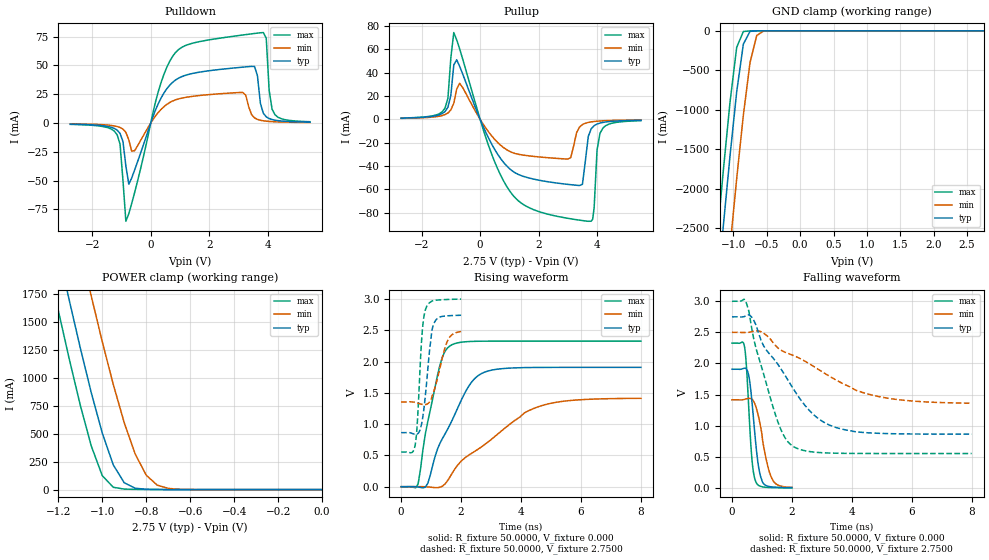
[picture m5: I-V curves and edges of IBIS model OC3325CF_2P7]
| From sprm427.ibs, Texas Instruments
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|   Model OC3325CF_2P7
[Model]   OC3325CF_2P7
Model_type   3-state
Polarity   Non-Inverting
Enable   Active-Low
Vmeas =   1.2500V
Cref =  15.0000pF
Rref = 100.0000M
Vref =  0.000V
C_comp   3.2189pF   3.2468pF   3.2081pF
[Temperature Range]   25.0000   0.1250k   -40.0000
[Pullup Reference]   2.7500V   2.5000V   3.0000V
[Pulldown Reference]   0.000V   0.000V   0.000V
[POWER Clamp Reference]   2.7500V   2.5000V   3.0000V
[GND Clamp Reference]   0.000V   0.000V   0.000V
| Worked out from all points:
|   slope of the pulldown table from 0 to 0.412 V, typ, clamps not added: 16.9 ohm
|   slope of the pullup table from 0 to 0.412 V, typ, clamps not added: 18.8 ohm
|   GND clamp passes 1 mA (typ) near -0.66 V on its own axis
|   POWER clamp passes 1 mA (typ) near -0.74 V on its own axis
|   rising waveform, R_fixture 50.0000, V_fixture 0.000: 20-80 % time 1.08ns typ, 2.21ns min, 559ps max; typ from 0 V to 1.91 V
|   rising waveform, R_fixture 50.0000, V_fixture 2.7500: 20-80 % time 237ps typ, 359ps min, 167ps max; typ from 0.864 V to 2.74 V
|   falling waveform, R_fixture 50.0000, V_fixture 0.000: 20-80 % time 236ps typ, 337ps min, 171ps max; typ from 1.91 V to 0.004 V
|   falling waveform, R_fixture 50.0000, V_fixture 2.7500: 20-80 % time 1.62ns typ, 2.58ns min, 864ps max; typ from 2.75 V to 0.864 V
[Pulldown]
| voltage   I(typ)   I(min)   I(max)
-2.75V    -942uA     -650uA     -1.14mA
-1.15V    -6.093mA   -2.984mA   -10.11mA
-850mV    -37.31mA   -8.054mA   -85.32mA
-550mV    -40.73mA   -24.01mA   -60.28mA
350mV     21.58mA    11.77mA    34.96mA
1.05V     40.19mA    21.58mA    65.58mA
3.15V     48.55mA    26.51mA    76.47mA
3.55V     49.14mA    4.497mA    77.79mA
3.85V     8.53mA     1.96mA     78.58mA
3.95V     5.417mA    1.638mA    73.77mA
4.15V     3.05mA     1.228mA    12mA
5.45V     763uA      461uA      1.156mA
[Pullup]
| voltage   I(typ)   I(min)   I(max)
-2.7V     968uA      800uA      1.062mA
-1.2V     6.635mA    4.013mA    9.529mA
-900mV    46.54mA    13.78mA    74.18mA
-700mV    45.39mA    30.78mA    60.33mA
1V        -42.09mA   -27.31mA   -60.87mA
3V        -55.65mA   -33.97mA   -84.69mA
3.4V      -56.64mA   -6.606mA   -86.26mA
3.7V      -14.62mA   -2.67mA    -87.25mA
3.85V     -6.777mA   -2.043mA   -85.39mA
4V        -4.07mA    -1.633mA   -26.14mA
4.1V      -3.234mA   -1.443mA   -12mA
5.5V      -811uA     -542uA     -1.184mA
[GND_clamp]
| voltage   I(typ)   I(min)   I(max)
-2.75V    -17.96A    -19.08A    -17.31A
-1.25V    -3.392A    -4.569A    -2.686A
-1.15V    -2.474A    -3.647A    -1.77A
-1.05V    -1.588A    -2.744A    -906.5mA
-950mV    -773.3mA   -1.875A    -209.6mA
-850mV    -168.3mA   -1.068A    -8.729mA
-750mV    -7.147mA   -403.1mA   -820uA
-650mV    -228.1uA   -59.73mA   -58.94uA
-550mV    -10.2uA    -3.869mA   -2.566uA
2.75V     178.5pA    235nA      161.8pA
[POWER_clamp]
| voltage   I(typ)   I(min)   I(max)
-2.75V    17.1A      17.93A     16.63A
-1.25V    2.586A     3.492A     2.054A
-1.2V     2.135A     3.04A      1.604A
-1.15V    1.695A     2.594A     1.168A
-1.05V    867.5mA    1.733A     390.3mA
-1V       506.5mA    1.325A     124.9mA
-950mV    221.4mA    942.3mA    20.88mA
-900mV    61.07mA    598.5mA    4.539mA
-850mV    12.29mA    317.3mA    2.127mA
-800mV    3.014mA    129mA      1.191mA
-750mV    1.14mA     39.91mA    598.9uA
0V        178.5pA    1.29nA     191.1pA
[Ramp]
| variable   typ   min   max
dV/dt_r   0.8390/0.7299n   0.2509/0.3309n   1.3849/0.5470n
dV/dt_f   0.6839/0.8576n   0.2184/0.4442n   1.3951/0.7940n
R_load = 50.0000
[Rising Waveform]
R_fixture = 50.0000
V_fixture = 0.000
V_fixture_min = 0.000
V_fixture_max = 0.000
| time   V(typ)   V(min)   V(max)
0s        1.106nV    5.188nV    804.6pV
565.7ps   -4.762mV   1.146mV    42.85mV
888.9ps   53.39mV    -3.639mV   1.041V
1.212ns   600.3mV    -15.26mV   1.778V
1.374ns   766mV      7.538mV    2.068V
1.616ns   978.4mV    146.9mV    2.246V
2.343ns   1.667V     530.9mV    2.321V
2.909ns   1.85V      717.9mV    2.326V
4.768ns   1.906V     1.306V     2.327V
8ns       1.907V     1.412V     2.327V
[Rising Waveform]
R_fixture = 50.0000
V_fixture = 2.7500
V_fixture_min = 2.5000
V_fixture_max = 3.0000
| time   V(typ)   V(min)   V(max)
0s        863.9mV    1.353V     553.4mV
363.6ps   851.4mV    1.355V     547.9mV
464.6ps   835.6mV    1.347V     656.5mV
545.5ps   843.1mV    1.337V     1.066V
707.1ps   1.068V     1.315V     2.496V
828.3ps   1.554V     1.314V     2.854V
1.01ns    2.432V     1.413V     2.961V
1.111ns   2.625V     1.555V     2.977V
1.556ns   2.731V     2.339V     2.992V
2ns       2.74V      2.479V     2.997V
[Falling Waveform]
R_fixture = 50.0000
V_fixture = 0.000
V_fixture_min = 0.000
V_fixture_max = 0.000
| time   V(typ)   V(min)   V(max)
0s        1.907V     1.416V     2.327V
424.2ps   1.925V     1.425V     2.254V
484.8ps   1.908V     1.432V     1.934V
545.5ps   1.836V     1.438V     1.418V
646.5ps   1.485V     1.431V     574.7mV
787.9ps   743.3mV    1.319V     108mV
888.9ps   334.8mV    1.138V     40.59mV
1.01ns    106.2mV    814.9mV    18.74mV
1.313ns   17.32mV    171.3mV    6.074mV
2ns       4.493mV    9.398mV    1.605mV
[Falling Waveform]
R_fixture = 50.0000
V_fixture = 2.7500
V_fixture_min = 2.5000
V_fixture_max = 3.0000
| time   V(typ)   V(min)   V(max)
0s        2.75V      2.5V       3V
484.8ps   2.772V     2.498V     2.966V
808.1ps   2.61V      2.525V     2.233V
1.051ns   2.288V     2.488V     1.839V
1.455ns   2.037V     2.287V     1.17V
2.02ns    1.613V     2.134V     674.4mV
2.748ns   1.168V     1.946V     575.9mV
3.556ns   959.3mV    1.713V     557.4mV
5.172ns   873.8mV    1.444V     553.6mV
8ns       864.2mV    1.361V     553.4mV
